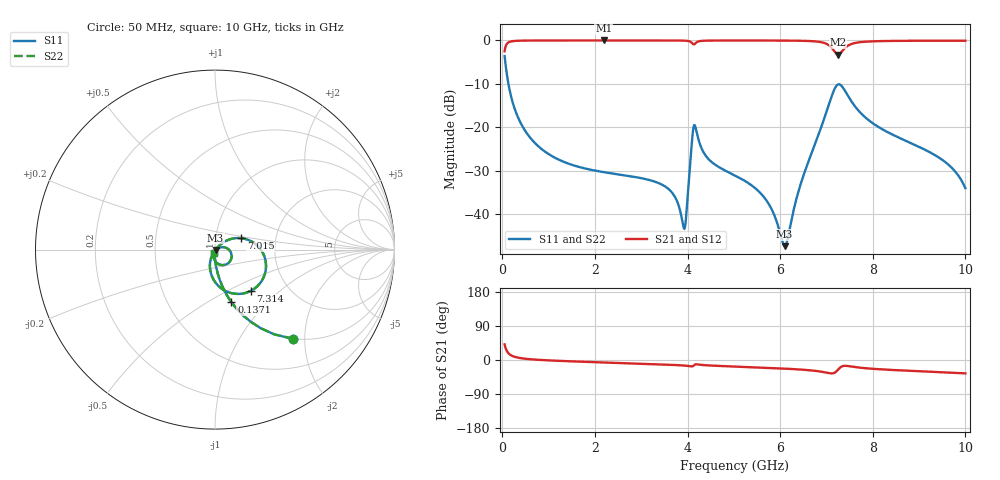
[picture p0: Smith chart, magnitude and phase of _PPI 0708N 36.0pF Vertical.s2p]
! S-Parameter data specifications (vertical orientation):
! Substrate: 40-mil Rogers 3003C, Substrate thickness, H=1.016mm, Dielectric constant, Er=3, Conductor thickness, T_mtl=0.043mm, Loss Tangent, Tand=0.003
! PCB Mounting Pad Footprint: Pad width, PadW=2.54mm , Pad length, PadL=0.51mm , Pad gap, PadG (edge-to-edge)=0.71mm , Reference planes=1.73mm apart
! Created Tue Jan 16 08:53:14 2018
# GHz S MA R 50
! 2 Port Network Data from SP1.SP block
! freq  magS11  angS11  magS21  angS21  magS12  angS12  magS22  angS22
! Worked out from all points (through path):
!   801 points, 50 MHz to 10 GHz, reference 50 ohm
!   highest |S21| = -0.01 dB at 2.189 GHz (marker M1); lowest = -3.2 dB at 7.251 GHz (marker M2)
!   group delay of S21, straight-line fit = 10.6 ps
!   lowest |S11| = -47.3 dB at 6.095 GHz (marker M3), VSWR 1.01, Z = 50.4 - j0.25 ohm
!   |S11| at or under -10 dB: 132.2 MHz to end of sweep
!   |S22| runs from -47.3 to -3.6 dB; largest |S21 - S12| = 0
!   S11 on the Smith chart (normalised r, x): 50 MHz: 0.99, -1.75; 137.1 MHz: 0.99, -0.64; 7.015 GHz: 1.33, +0.17; 7.314 GHz: 1.31, -0.66; 10 GHz: 0.99, -0.04
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0.05  0.6601 -48.9  0.751 41.1  0.751 41.1  0.6601 -48.9
0.1370625  0.3058 -72.7  0.9519 17.3  0.9519 17.3  0.3058 -72.7
0.3360625  0.1314 -83.6  0.9911 6.3  0.9911 6.3  0.1314 -83.6
0.647  0.07129 -88.2  0.9972 1.6  0.9972 1.6  0.07129 -88.2
1.716625  0.03439 -93.9  0.9989 -4.6  0.9989 -4.6  0.03439 -93.9
2.18925  0.03056 -95.7  0.999 -6.6  0.999 -6.6  0.03056 -95.7
3.370812  0.02291 -99.2  0.9987 -11.4  0.9987 -11.4  0.02291 -99.2
3.706625  0.01658 -96.8  0.9979 -13.1  0.9979 -13.1  0.01658 -96.8
3.9305  0.006796 -39.0  0.9936 -14.7  0.9936 -14.7  0.006796 -39.0
4.104625  0.07824 -0.5  0.9245 -16.7  0.9245 -16.7  0.07824 -0.5
4.166812  0.1026 -55.1  0.9228 -11.7  0.9228 -11.7  0.1026 -55.1
4.440437  0.04393 -98.6  0.9946 -14.2  0.9946 -14.2  0.04393 -98.6
5.025  0.02796 -103.7  0.9976 -17.3  0.9976 -17.3  0.02796 -103.7
5.684188  0.01494 -101.0  0.9972 -20.4  0.9972 -20.4  0.01494 -101.0
6.094625  0.004302 -35.2  0.9955 -22.7  0.9955 -22.7  0.004302 -35.2
6.691625  0.05282 42.1  0.9803 -27.8  0.9803 -27.8  0.05282 42.1
7.015  0.1593 23.5  0.9047 -33.8  0.9047 -33.8  0.1593 23.5
7.251313  0.3122 -30.4  0.6883 -25.3  0.6883 -25.3  0.3122 -30.4
7.3135  0.3047 -48.8  0.7251 -18.2  0.7251 -18.2  0.3047 -48.8
7.599563  0.1792 -90.2  0.9292 -18.3  0.9292 -18.3  0.1792 -90.2
8.345812  0.08673 -109.0  0.9857 -25.8  0.9857 -25.8  0.08673 -109.0
10  0.01994 -102.2  0.9916 -35.3  0.9916 -35.3  0.01994 -102.2
